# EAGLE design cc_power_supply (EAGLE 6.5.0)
REV: A; TITLE: Coilcube Power Supply
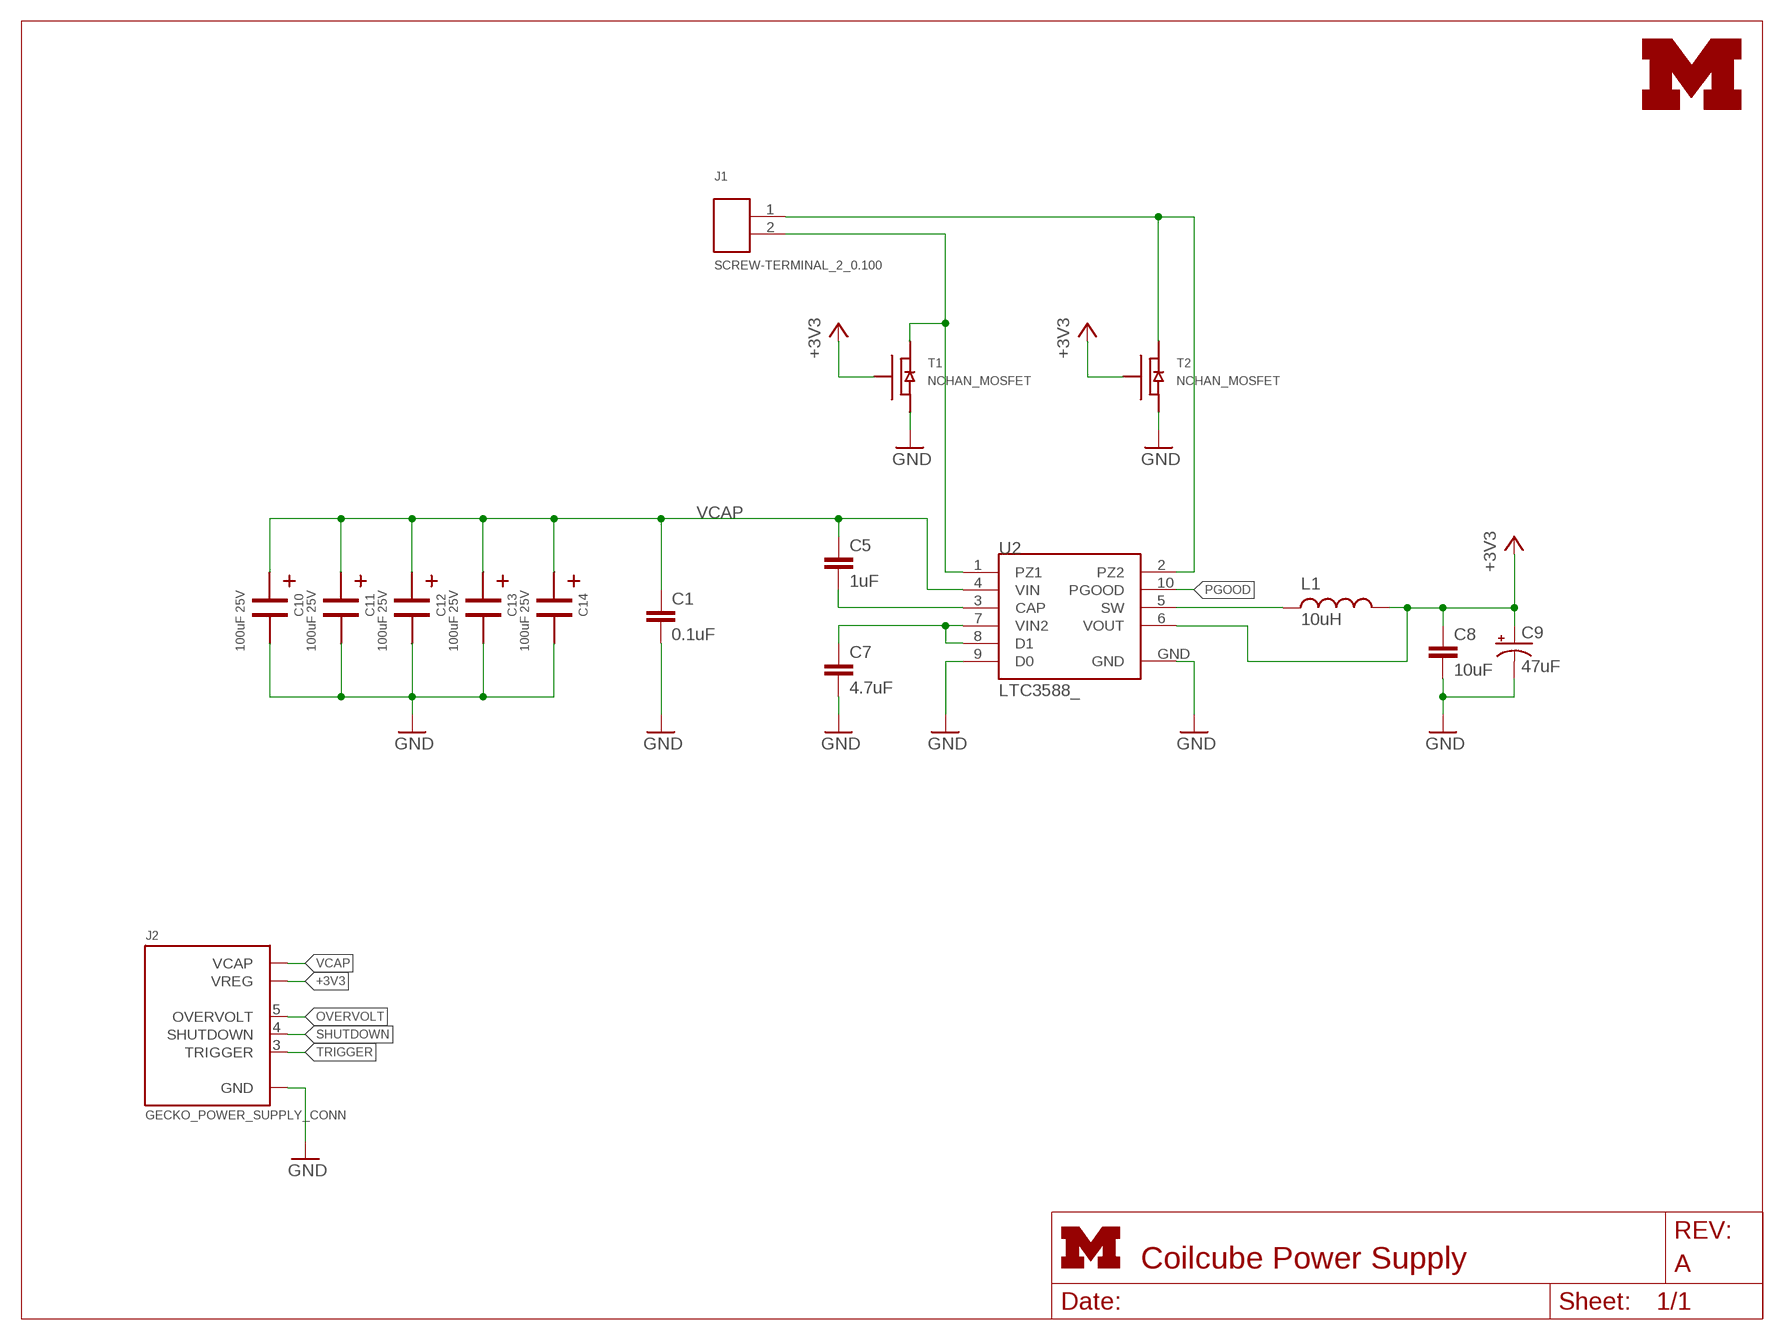
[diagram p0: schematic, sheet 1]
FRAME5 (LETTER_L): HEIGHT: 8.5in; WIDTH: 11in

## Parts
C1  0.1uF  C-EUC0603  [C0603]
C5  1uF  C-EUC0603  [C0603]
C7  4.7uF  C-EUC0603  [C0603]
C8  10uF  C-EUC1206  [C1206]
C9  47uF  CAP_POL1206  [EIA3216]
C10  100uF 25V  2917_CAP_POL  [2917_CAP_POL]
C11  100uF 25V  2917_CAP_POL  [2917_CAP_POL]
C12  100uF 25V  2917_CAP_POL  [2917_CAP_POL]
C13  100uF 25V  2917_CAP_POL  [2917_CAP_POL]
C14  100uF 25V  2917_CAP_POL  [2917_CAP_POL]
J1  SCREW-TERMINAL_2_0.100  [CONN_BLOCK_2]
J2  GECKO_POWER_SUPPLY_CONN  [HEADER1X6/0.05IN]
L1  10uH  INDUCTOR1210  [1210]
T1  NCHAN_MOSFET  [NCHAN_MOSFET]
T2  NCHAN_MOSFET  [NCHAN_MOSFET]
U2  LTC3588_  [MSOP-10-GNDPAD]
U$2  UMICH_SOLID_SMALL  [UMICH_SOLID_75MIL]

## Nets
+3V3: C8.1 C9.A(+) J2.2(VREG) L1.2 T1.G T2.G U2.6(VOUT)
GND: C1.2 C7.2 C8.2 C9.C(-) C10.- C11.- C12.- C13.- C14.- J2.1(GND) T1.S T2.S U2.9(D0) U2.GND
N$20: L1.1 U2.5(SW)
N$22: C5.2 U2.3(CAP)
OVERVOLT: J2.5(OVERVOLT)
PGOOD: U2.10(PGOOD)
PZ1: J1.2 T1.D U2.1(PZ1)
PZ2: J1.1 T2.D U2.2(PZ2)
SHUTDOWN: J2.4(SHUTDOWN)
TRIGGER: J2.3(TRIGGER)
VCAP: C1.1 C5.1 C10.+ C11.+ C12.+ C13.+ C14.+ J2.6(VCAP) U2.4(VIN)
VIN2: C7.1 U2.7(VIN2) U2.8(D1)

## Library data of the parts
C1 = rcl:C-EU: CAPACITOR, European symbol; DIGIKEY: 445-1316-1-ND
C5 = rcl:C-EU: CAPACITOR, European symbol; DIGIKEY: 445-1321-1-ND
C7 = rcl:C-EU: CAPACITOR, European symbol; DIGIKEY: 445-5178-1-ND
C8 = rcl:C-EU: CAPACITOR, European symbol; DIGIKEY: 399-8152-1-ND
C9 = SparkFun-Passives:CAP_POL: Capacitor Polarized; DIGIKEY: 399-3700-1-ND
C10-C14 = coilcube:2917_CAP_POL; DIGIKEY: 399-5175-1-ND
J1 = headers:SCREW-TERMINAL_2_0.100: 2x 0.100 in screw terminal block; DIGIKEY: 277-1273-ND
J2 = gecko:GECKO_POWER_SUPPLY_CONN: Header on the gecko power supply board.
L1 = SparkFun-Passives:INDUCTOR: Inductors; DIGIKEY: 587-1625-1-ND
T1 T2 = Power_Metering:NCHAN_MOSFET; DIGIKEY: SI1302DL-T1-GE3CT-ND
U2 = SparkFun-PowerIC:LTC3588: Energy Harvesting Power Supply; DIGIKEY: LTC3588EMSE-1#PBF-ND
U$2 = logos:UMICH_SOLID

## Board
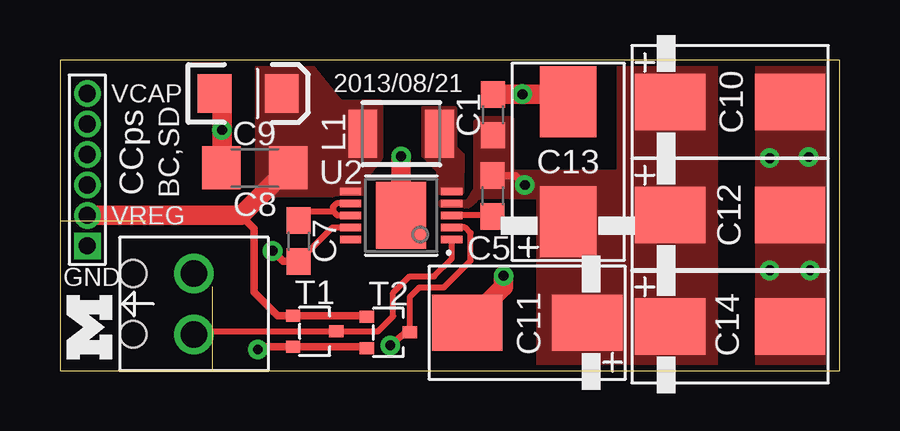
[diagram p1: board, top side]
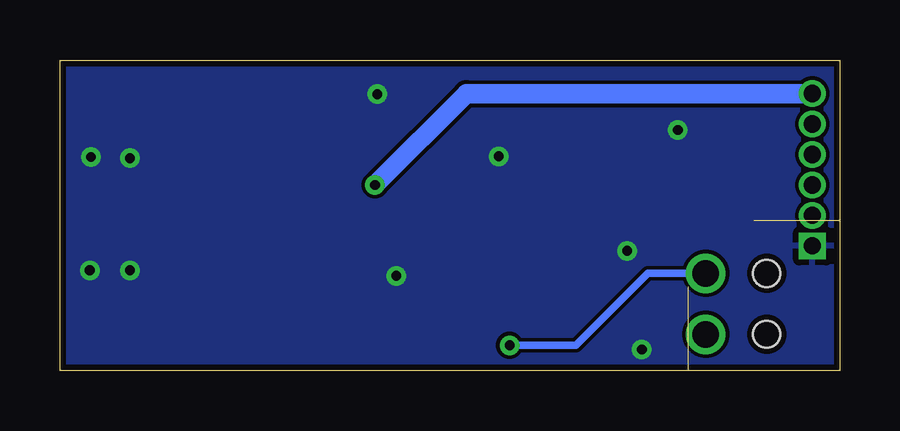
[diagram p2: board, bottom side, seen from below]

Size 32.51 x 12.95 mm. Coordinates in mm from the lower left corner, seen from the top.
Outline: 0,0 32.51,0 32.51,12.95 0,12.95 0,0
Copper layers (1*16): Top 0.0178mm / dielectric 59mil / Bottom 0.0178mm
Design rules "sunstone-2lyr_v1.0.0.3 *": minimum track width 6mil, minimum drill 14mil, track to track 6mil, track to pad 6mil, pad to pad 6mil, via to via 6mil, smd to smd 6mil, copper to edge 10mil, drill to drill 16mil, minimum pad ring 8mil, minimum via ring 8mil, stop-mask expansion 3mil, vias tented up to drill 20mil, thermal gap 10mil
Milling: 2 lines

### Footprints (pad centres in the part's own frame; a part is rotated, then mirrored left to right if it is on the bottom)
C0603 = smd 1.1 x 1: 1 -0.85,0; 2 0.85,0
C1206 = smd 1.6 x 1.8: 1 -1.4,0; 2 1.4,0
EIA3216 = smd 1.4 x 1.6: A 1.4,0; C -1.4,0
2917_CAP_POL = smd 2.95 x 2.35: + -2.5,0; - 2.5,0
CONN_BLOCK_2 = drill 1.1: 1 -1.27,0; 2 1.27,0 | hole 1.12: -1.27,-2.54; 1.27,-2.54
HEADER1X6/0.05IN = drill 0.711 pad 1.016 square: 1 -2.54,0 | drill 0.711 pad 1.016: 2 -1.27,0; 3 0,0; 4 1.27,0; 5 2.54,0; 6 3.81,0
1210 = smd 1.2 x 2: 1 -1.6,0; 2 1.6,0
NCHAN_MOSFET = smd 0.6 x 0.5: D -0.9,0; G 0.9,-0.65; S 0.9,0.65
MSOP-10-GNDPAD = smd 0.305 x 0.889: 1 -1,-2.11; 2 -0.5,-2.11; 3 0,-2.11; 4 0.5,-2.11; 5 1,-2.11; 6 1,2.11; 7 0.5,2.11; 8 0,2.11; 9 -0.5,2.11; 10 -1,2.11 | smd 2.794 x 2.083: GND 0,0

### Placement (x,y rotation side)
C1  18.06,10.67 90 top
C5  18.03,7.29 270 top
C7  9.94,5.41 270 top
C8  8.13,8.46 180 top
C9  7.85,11.56 0 top
C10  27.94,11.2 0 top
C11  19.48,2.01 180 top
C12  27.94,6.5 0 top
C13  21.18,8.71 90 top
C14  27.94,1.85 0 top
J1  5.59,2.79 270 top
J2  1.14,7.75 90 top
L1  14.22,9.88 180 top
T1  10.62,1.65 180 top
T2  13.69,1.6 180 top
U2  14.22,6.48 90 top
U$2  2.18,0.48 90 top

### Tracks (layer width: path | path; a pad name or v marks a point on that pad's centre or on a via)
+3V3
  Top 0.254: T2.G 12.74,2.3
  Top 0.305: 12.74,2.3 T1.G 9.08,2.3 8.1,3.28 8.1,5.92 7.55,6.48
  Top 0.813: J2.2 7.55,6.48 C8.1
  pour Top (no thermals): 8.26,12.7 10.46,12.67 11.66,11.2 13.34,11.2 13.34,8.89 12.62,7.95 12.62,7.34 8.26,7.34
GND  (via drill 0.41 pad 0.3)
  Top 0.254: C7.2 11.36,5.98 U2.9
  Top 0.305: T2.S 12.74,1 T1.S 8.37,1 v8.26,0.89 | C7.2 9.31,4.56 v8.87,5
  Top 0.813: C11.- 18.49,3.52 v18.49,3.96 | C13.- 20.95,11.52 19.29,11.52 v19.28,11.53 18.07,11.53 C1.2 | U2.GND v14.22,8.94 | C8.2 6.75,8.48 v6.75,10.03 v6.76,10.03 v6.75,10.04 6.75,11.25 C9.C
  other vias: 29.59,8.86 31.22,8.92 31.27,4.19 29.59,4.19
  pour Top (rank 5, no thermals): 29.11,12.93 31.8,12.93 31.8,-0.03 29.11,-0.03
  pour Bottom: -0.64,13.34 33.02,13.34 33.02,-0.64 -0.64,-0.64
N$20
  pour Top (no thermals): 15.79,7.45 16.74,7.45 16.76,8.97 16.45,9.28 16.45,10.91 15.18,10.91 15.18,9 15.81,8.37
N$22
  Top 0.254: C5.2 18,6.48 U2.3
PZ1
  Top 0.254: J1.2 5.71,1.65 T1.D 13.26,1.65 13.89,2.29 13.89,3.25 14.58,3.94 15.6,3.94 16.33,4.67 U2.1
PZ2  (via drill 0.41 pad 0.3)
  Top 0.254: T2.D 14.59,3.08 14.99,3.48 16,3.48 17.12,4.6 17.12,5.74 16.88,5.98 U2.2
  Top 0.305: T2.D 14.43,1.6 v13.77,1.07
  Bottom 0.305: J1.1 8,4.06 11,1.07 v13.77,1.07
VCAP  (via drill 0.41 pad 0.3)
  Top 0.305: v19.38,7.75 18.99,8.14 C5.1
  Bottom 0.813: v19.38,7.75 15.57,11.56 J2.6
  pour Top (no thermals): 27.33,12.95 23.32,12.95 23.32,8.26 18.82,8.26 18.82,10.49 17.48,10.49 17.48,10.36 17.35,10.36 17.35,7.57 16.99,7.01 15.9,7.01 15.9,6.91 17.04,6.91 17.5,7.29 19.96,7.26 19.96,0.03 27.33,0.03
VIN2
  Top 0.254: U2.7 11.52,6.98 11.38,6.83 11.38,6.66 | 11.38,6.66 11.56,6.48 U2.8 | C7.1 10.34,6.66 11.38,6.66

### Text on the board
tPlace: VCAP | 2013/08/21 | CCps | BC,SD | VREG | GND

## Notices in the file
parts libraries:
SparkFun-PowerIC: Licensing: CC v3.0 Share-Alike You are welcome to use this library for commercial purposes.
